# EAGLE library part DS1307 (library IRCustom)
DS1307 Real time clock (RTC) with battery backup ability. Talk to it via i2c
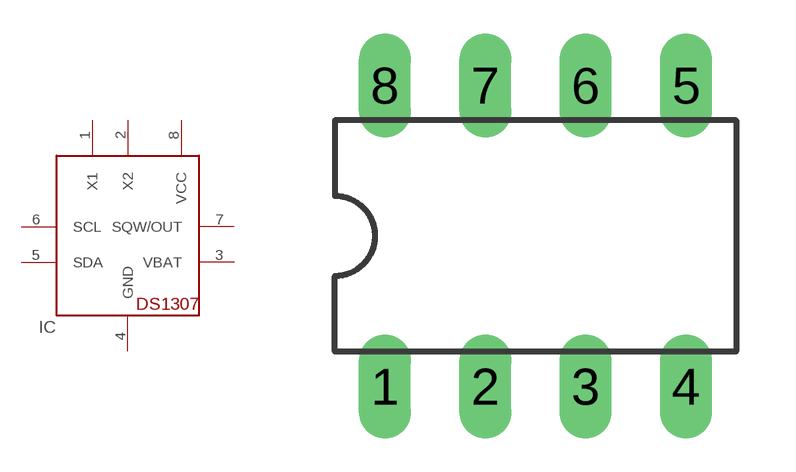
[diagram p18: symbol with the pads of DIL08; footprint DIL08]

Designator prefix IC

## DS1307  [DIL08]
1  X1  pas
2  X2  pas
3  VBAT  pwr
4  GND  pwr
5  SDA
6  SCL
7  SQW/OUT
8  VCC  pwr

## Footprint DIL08 (pad centres in mm)
Dual In Line Package
drill 0.813 long: 1 -3.81,-3.81; 2 -1.27,-3.81; 3 1.27,-3.81; 4 3.81,-3.81; 5 3.81,3.81; 6 1.27,3.81; 7 -1.27,3.81; 8 -3.81,3.81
